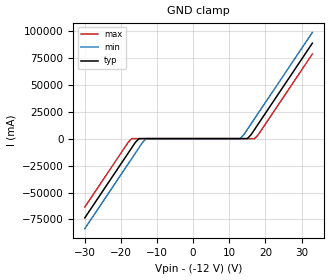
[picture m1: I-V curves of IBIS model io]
| TEXAS INSTRUMENTS INCORPORATED
| 2 Channel-Bi-directional SURGE-ESD Protection Device
| Marketing Part #   Voltage Range   Package-type   #pins/pkg drawing
| ESD862   -12V-12V   SOT   3/DBZ
[IBIS Ver]   4.1
[Comment char]  |_char
[File Name]   esds552.ibs
[File Rev]   1.0
"[Date]   Jan 15, 2024 "
[Source]   Data created from TI-SPICE simulations at TI-SLL/HVL.
   The following is an IBIS list for the ESDS552.
   Please contact sllibis@ti.com with questions and
   comments concerning SLL IBIS models.
[Notes]
   - New measurements under nominal conditions only.
[Disclaimer]
"| TI and its licensors and suppliers make no warranties, either expressed"
"| or implied, with respect to this  model, including the warranties of "
"| provided solely on an ""as is"" basis. The entire risk as to its quality "
| and performance is with the customer.
[Copyright]
| (C) Copyright 2024 Texas Instruments Incorporated. All rights reserved.
| Component ESDS552_DBZ 3-PIN SOT
[Component]   ESDS552_DBZ
"[Manufacturer]   Texas Instruments, Inc."
[Package]   |3 SOT - DBZ package
   typ   min   max
R_pkg   74.0E-03   54.0E-03   94.0E-03
L_pkg   9.0E-10   7.0E-10   11.0E-10
C_pkg   8.5E-13   6.50E-13   10.50E-13
[Pin]   signal_name   model_name   R_pin   L_pin   C_pin
1   IO   io   2.07E-03   2.09E-10   6.95E-14
2   IO   io   2.07E-03   2.09E-10   6.95E-14
3   GND   gnd   2.07E-03   2.09E-10   6.95E-14
| Models and submodels in the file (1): io (Input)
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|   io Model
[Model]   io
Model_type  Input
| variable   typ   min   max
C_comp   9.5pF   8.5pF   10.5pF
[Voltage Range]   24   20   28
[Temperature Range]   27   -55   150
[Power Clamp Reference]   0   0   0
[GND Clamp Reference]   -12   -10   -14
[GND Clamp]
|	Voltage  I(typ)   I(min)   I(max)
-30V      -73.5A     -83.5A     -63.5A
-18V      -13.5A     -23.5A     -3.5A
-17V      -8.5A      -18.5A     -11.1nA
-16V      -3.5A      -13.5A     -10.5nA
-15V      -9.8nA     -8.5A      -9.8nA
-13V      -8.5nA     -8.5nA     -8.5nA
13V       8.5nA      8.5nA      8.5nA
15V       9.8nA      8.5A       9.8nA
16V       3.5A       13.5A      10.5nA
17V       8.5A       18.5A      11.1nA
18V       13.5A      23.5A      3.5A
33V       88.5A      98.5A      78.5A
[Power Clamp]
|   Voltage   I(typ)   I(min)   I(max)
-12V      0A         0A         0A
0V        0A         0A         0A
12V       0A         0A         0A
